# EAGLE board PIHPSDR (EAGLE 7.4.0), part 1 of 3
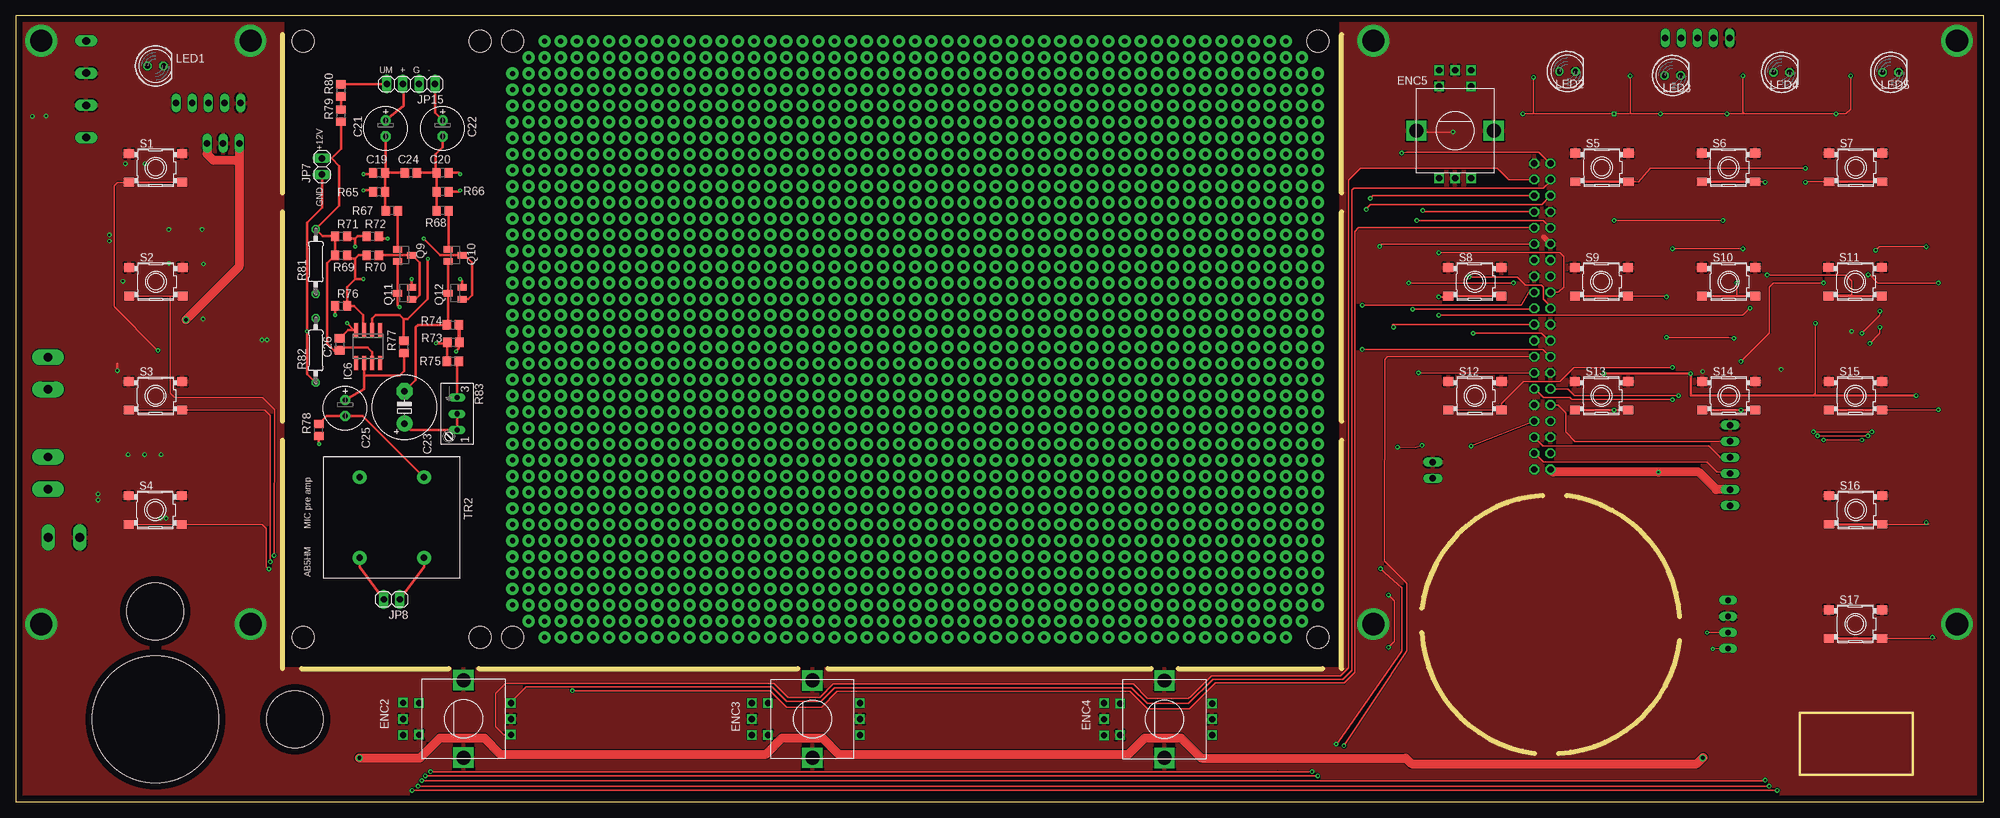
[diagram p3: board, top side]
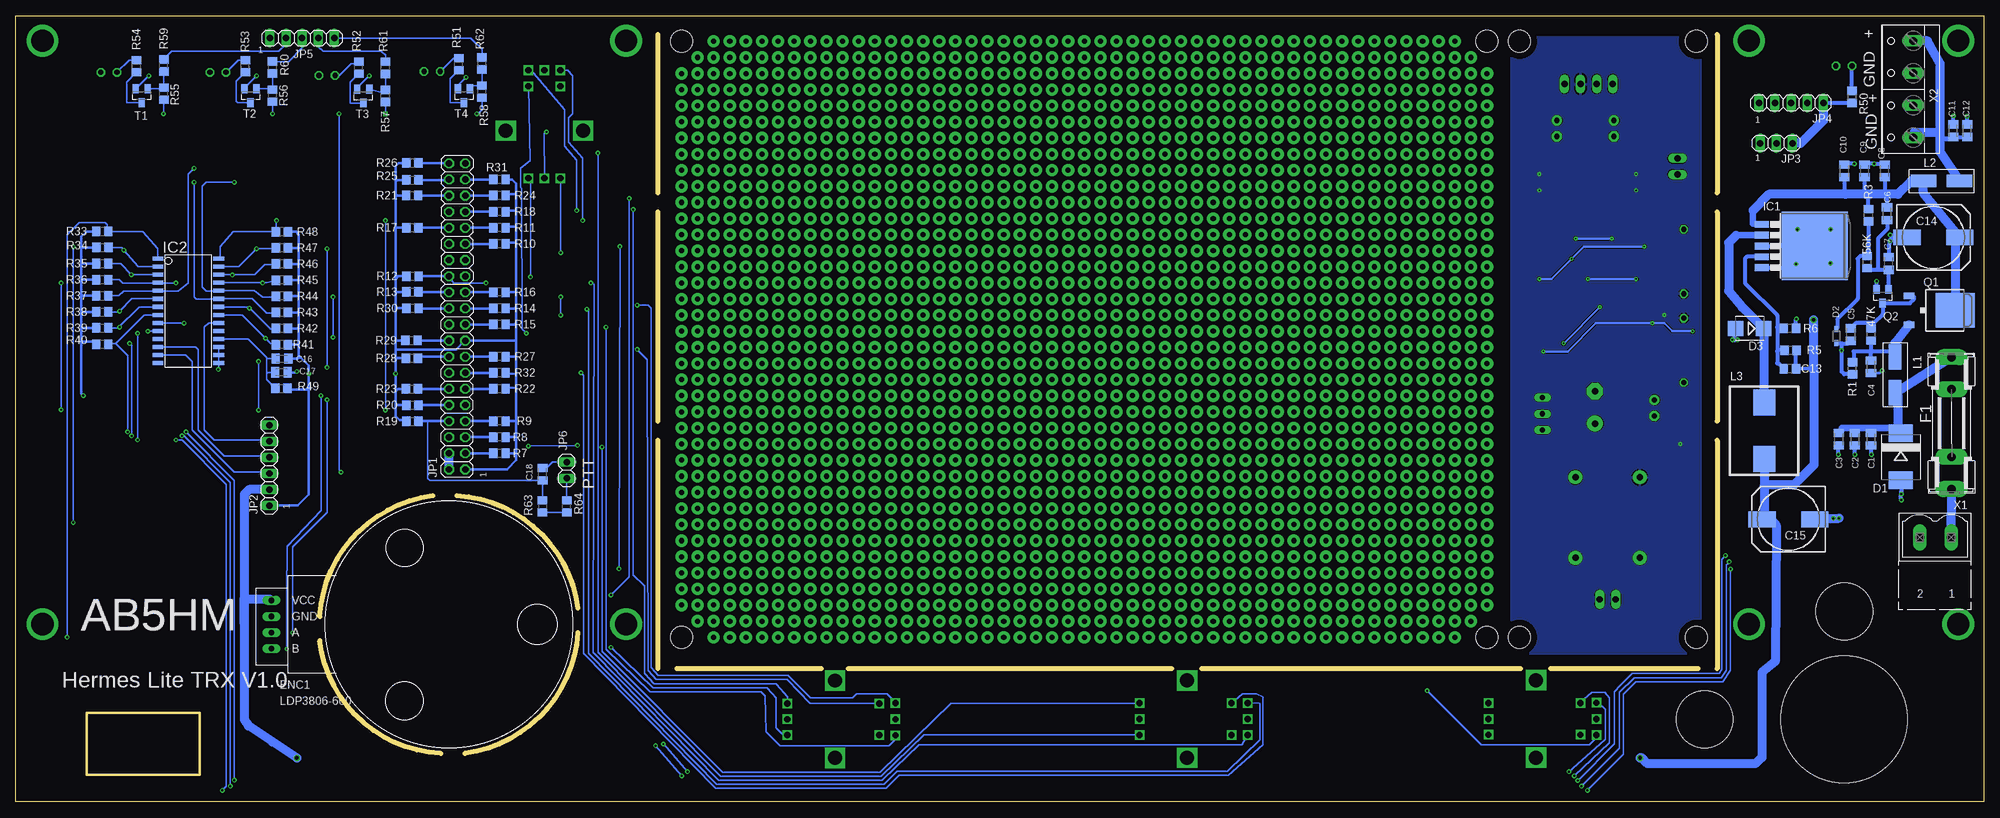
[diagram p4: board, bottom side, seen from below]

Size 310.21 x 123.94 mm. Coordinates in mm from the lower left corner, seen from the top.
Outline: 0,0 310.21,0 310.21,123.94 0,123.94 0,0
Copper layers (1*16): Top 0.035mm / dielectric 1.5mm / Bottom 0.035mm
Design rules "default *": minimum track width 10mil, minimum drill 0.19811875mm, track to track 4mil, track to pad 4mil, pad to pad 4mil, via to via 4mil, smd to smd 6mil, copper to edge 40mil, drill to drill 8mil, minimum pad ring 10mil, minimum via ring 8mil, stop-mask expansion 4mil, vias tented up to drill 0mil, thermal gap 10mil
Holes 9 mm at 22,30 44,13
Holes 20 mm at 22,13
Holes 3.5 mm at 45.26,119.92 73.2,119.92 78.28,119.92 205.28,119.92 205.28,25.94 78.28,25.94 73.2,25.94 45.26,25.94
Milling: 14 lines

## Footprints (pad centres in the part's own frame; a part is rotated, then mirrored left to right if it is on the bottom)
R0805 = smd 1.3 x 1.5: 1 -0.95,0; 2 0.95,0
C0805K = smd 1.3 x 1.6: 1 -1,0; 2 1,0
C0805 = smd 1.3 x 1.5: 1 -0.95,0; 2 0.95,0
140CLH-1010 = smd 4.3 x 2.5: + 4.15,0; - -4.15,0
E2,5-7 = drill 0.813 pad 1.6: + -1.27,0 | drill 0.813 pad 1.6 octagon: - 1.27,0
E5-10,5 = drill 1.016 pad 2.54: + -2.54,0 | drill 1.016 pad 2.54 octagon: - 2.54,0
SMC = smd 2.8 x 3.8: A 3.7,0; C -3.7,0
SOD323 = smd 1 x 0.6: 1 -1.1,0; 2 1.1,0
SMB = smd 2.4 x 2.4: A 2.2,0; C -2.2,0
LPD3806_ROTARY = drill 0.9 long: A -27.94,-1.27; B -27.94,-3.81; GND -27.94,1.27; VCC -27.94,3.81
ALPS_EC11E_SW = drill 1 square: A -2.5,-7.5; A' -2.54,9.525; B 2.5,-7.5; B' 2.54,9.525; C 0,-7.5; C' 0,9.525; D -2.5,7; E 2.5,7 | drill 2.2 square: GND1 -6.1,0; GND2 6.1,0
SHK20L = drill 1.321 pad 2.54 long: 1A -10.414,0; 1B -5.334,0; 2A 10.414,0; 2B 5.334,0
TO263-5 = smd 1.067 x 2.159: 1 -3.404,-5.791; 2 -1.702,-5.791; 3 0,-5.791; 4 1.702,-5.791; 5 3.404,-5.791 | smd 10.8 x 10.41: 6 0,2.54
SO28W = smd 0.65 x 1.7: 1 -7.62,-4.78; 2 -6.35,-4.78; 3 -5.08,-4.78; 4 -3.81,-4.78; 5 -2.54,-4.78; 6 -1.27,-4.78; 7 0,-4.78; 8 1.27,-4.78; 9 2.54,-4.78; 10 3.81,-4.78; 11 5.08,-4.78; 12 6.35,-4.78; 13 7.62,-4.78; 14 8.89,-4.78; 15 8.89,4.78; 16 7.62,4.78; 17 6.35,4.78; 18 5.08,4.78; 19 3.81,4.78; 20 2.54,4.78; 21 1.27,4.78; 22 0,4.78; 23 -1.27,4.78; 24 -2.54,4.78; 25 -3.81,4.78; 26 -5.08,4.78; 27 -6.35,4.78; 28 -7.62,4.78
SO8 = smd 0.6 x 2.2: 1 -1.905,-2.6; 2 -0.635,-2.6; 3 0.635,-2.6; 4 1.905,-2.6; 5 1.905,2.6; 6 0.635,2.6; 7 -0.635,2.6; 8 -1.905,2.6
2X20 = drill 1.016 octagon: 1 -24.13,-1.27; 2 -24.13,1.27; 3 -21.59,-1.27; 4 -21.59,1.27; 5 -19.05,-1.27; 6 -19.05,1.27; 7 -16.51,-1.27; 8 -16.51,1.27; 9 -13.97,-1.27; 10 -13.97,1.27; 11 -11.43,-1.27; 12 -11.43,1.27; 13 -8.89,-1.27; 14 -8.89,1.27; 15 -6.35,-1.27; 16 -6.35,1.27; 17 -3.81,-1.27; 18 -3.81,1.27; 19 -1.27,-1.27; 20 -1.27,1.27; 21 1.27,-1.27; 22 1.27,1.27; 23 3.81,-1.27; 24 3.81,1.27; 25 6.35,-1.27; 26 6.35,1.27; 27 8.89,-1.27; 28 8.89,1.27; 29 11.43,-1.27; 30 11.43,1.27; 31 13.97,-1.27; 32 13.97,1.27; 33 16.51,-1.27; 34 16.51,1.27; 35 19.05,-1.27; 36 19.05,1.27; 37 21.59,-1.27; 38 21.59,1.27; 39 24.13,-1.27; 40 24.13,1.27
1X06 = drill 1.016 long: 1 -6.35,0; 2 -3.81,0; 3 -1.27,0; 4 1.27,0; 5 3.81,0; 6 6.35,0
1X03 = drill 1.016 long: 1 -2.54,0; 2 0,0; 3 2.54,0
1X05 = drill 1.016 long: 1 -5.08,0; 2 -2.54,0; 3 0,0; 4 2.54,0; 5 5.08,0
1X02 = drill 1.016 long: 1 -1.27,0; 2 1.27,0
1X04 = drill 1.016 long: 1 -3.81,0; 2 -1.27,0; 3 1.27,0; 4 3.81,0
SM_BEAD = smd 4 x 2: P$1 -2.857,0; P$2 2.857,0
PULSE_PA4342 = smd 3.5 x 4.1: 1 0,4.445; 2 0,-4.445
LED5MM = drill 0.813 octagon: A -1.27,0; K 1.27,0
TO252 = smd 1 x 1.6: 1 -2.28,-4.8; 2 2.28,-4.8 | smd 5.4 x 6.2: 3 0,2.5
SOT23 = smd 1 x 1.4: 1 -0.95,-1.1; 2 0.95,-1.1; 3 0,1.1
SOT23-BEC = smd 1 x 1.4: B -0.95,-1.1; C 0,1.1; E 0.95,-1.1
0207/10 = drill 0.813 octagon: 1 -5.08,0; 2 5.08,0
S64W = drill 0.813 long: A 2.54,1.27; E -2.54,1.27; S 0,1.27
TL3301-SMD = smd 1.6 x 1.4: 1 -4.2,2.25; 2 4.2,2.25; 3 -4.2,-2.25; 4 4.2,-2.25
SV1-500 = drill 1 pad 2.184: 1 -5.08,-6.35; 3 5.08,-6.35; 4 5.08,6.35; 6 -5.08,6.35
MSTBV2 = drill 1.397 long: 1 -2.5,0; 2 2.5,0
W237-4P = drill 1.194 long: 1 -7.62,-0.635; 2 -2.54,-0.635; 3 2.54,-0.635; 4 7.62,-0.635

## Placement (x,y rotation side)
47K  100k  [R0805]  17.76,73.68 270 bottom
56K  180k  [R0805]  18.39,85.11 270 bottom
C1  10u  [C0805K]  17.76,57.17 270 bottom
C2  10u  [C0805K]  20.3,57.17 270 bottom
C3  0.1u  [C0805K]  22.84,57.17 270 bottom
C4  10u  [C0805K]  17.76,68.6 270 bottom
C5  0.1u  [C0805K]  20.93,73.68 270 bottom
C6  10u  [C0805K]  15.22,92.73 270 bottom
C7  0.1u  [C0805K]  14.98,84.88 90 bottom
C8  10u  [C0805K]  15.61,99.48 90 bottom
C9  0.1u  [C0805K]  18.79,99.48 90 bottom
C10  0.1u  [C0805K]  21.96,99.48 90 bottom
C11  0.1u  [C0805K]  4.82,105.83 90 bottom
C12  0.1u  [C0805K]  2.59,105.83 90 bottom
C13  np  [C0805]  30.54,68.29 180 bottom
C14  220u  [140CLH-1010]  7.91,89 0 bottom
C15  220u  [140CLH-1010]  30.77,44.55 180 bottom
C16  10u  [C0805K]  268.26,69.88 180 bottom
C17  1n  [C0805K]  268.35,67.73 0 bottom
C18  100n  [C0805K]  227.19,51.66 90 bottom
C19  680p  [C0805]  57.27,99.19 180 top
C20  680p  [C0805]  67.27,99.19 180 top
C21  47/63  [E2,5-7]  58.27,106.19 270 top
C22  47/63  [E2,5-7]  67.27,106.19 270 top
C23  1000/6  [E5-10,5]  61.27,62.19 90 top
C24  330p  [C0805]  62.27,99.19 180 top
C25  47/63  [E2,5-7]  51.91,62.09 270 top
C26  0.1u  [C0805]  51.05,72.13 270 top
D1  [SMC]  13.07,54.4 270 bottom
D2  BAS16J  [SOD323]  23.23,73.45 90 bottom
D3  SS54B-HF  [SMB]  36.89,74.64 180 bottom
ENC1  LDP3806-600  [LPD3806_ROTARY]  241.96,27.96 0 bottom
ENC2  EC11E_SW  [ALPS_EC11E_SW]  70.57,13.07 90 top
ENC3  EC11E_SW  [ALPS_EC11E_SW]  125.57,13.04 90 top
ENC4  EC11E_SW  [ALPS_EC11E_SW]  181.07,13.01 90 top
ENC5  EC11E_SW  [ALPS_EC11E_SW]  226.89,105.84 0 top
F1  5A  [SHK20L]  5.06,59.71 90 bottom
IC1  LM2596S  [TO263-5]  29.19,87.65 270 bottom
IC2  MCP23017SO  [SO28W]  283.03,78.05 270 bottom
IC6  TL071  [SO8]  55.54,71.83 180 top
JP1  [2X20]  240.65,76.54 90 bottom
JP2  [1X06]  270.25,53.04 90 bottom
JP3  [1X03]  32.67,103.85 180 bottom
JP4  [1X05]  30.34,110.2 180 bottom
JP5  [1X05]  265.08,120.43 0 bottom
JP6  PTT  [1X02]  223.38,52.29 90 bottom
JP7  [1X02]  48.27,100.19 90 top
JP8  [1X02]  59.27,31.92 180 top
JP15  [1X04]  62.27,113.19 180 top
L1  2743021447  [SM_BEAD]  13.95,67.33 90 bottom
L2  2743021447  [SM_BEAD]  6.64,97.89 0 bottom
L3  47uH  [PULSE_PA4342]  34.58,58.52 0 bottom
LED1  [LED5MM]  22.02,116.04 0 top
LED2  [LED5MM]  244.59,115.17 0 top
LED3  [LED5MM]  261.16,114.53 0 top
LED4  [LED5MM]  278.36,115.03 0 top
LED5  [LED5MM]  295.55,115.03 0 top
Q1  FDD6685  [TO252]  6.96,77.49 270 bottom
Q2  IRLM6244  [SOT23]  15.93,79.72 180 bottom
Q9  BC847A  [SOT23]  61.27,86.19 270 top
Q10  BC847A  [SOT23]  69.27,86.19 270 top
Q11  BC858A  [SOT23-BEC]  61.27,80.19 90 top
Q12  BC858A  [SOT23-BEC]  69.27,80.19 90 top
R1  10k  [R0805]  20.69,68.37 90 bottom
R3  100k  [R0805]  18.15,92.5 90 bottom
R5  3K05  [R0805]  30.45,71.22 0 bottom
R6  1k  [R0805]  30.54,74.64 180 bottom
R7  10k  [R0805]  233.97,54.95 180 bottom
R8  10k  [R0805]  233.97,57.49 180 bottom
R9  10k  [R0805]  233.97,60.03 180 bottom
R10  10k  [R0805]  233.97,87.97 180 bottom
R11  10  [R0805]  233.97,90.52 180 bottom
R12  10k  [R0805]  247.68,82.89 0 bottom
R13  10k  [R0805]  247.69,80.4 0 bottom
R14  10k  [R0805]  233.97,77.81 180 bottom
R15  10k  [R0805]  233.97,75.28 180 bottom
R16  10k  [R0805]  233.97,80.36 180 bottom
R17  10k  [R0805]  247.71,90.54 0 bottom
R18  10k  [R0805]  233.97,93.06 180 bottom
R19  10k  [R0805]  247.71,60 0 bottom
R20  10k  [R0805]  247.71,62.57 0 bottom
R21  10k  [R0805]  247.73,95.62 0 bottom
R22  10k  [R0805]  233.97,65.11 180 bottom
R23  10k  [R0805]  247.77,65.11 0 bottom
R24  10k  [R0805]  233.97,95.59 180 bottom
R25  10k  [R0805]  247.71,98.05 0 bottom
R26  10k  [R0805]  247.71,100.75 0 bottom
R27  10k  [R0805]  233.97,70.19 180 bottom
R28  10k  [R0805]  247.79,69.95 0 bottom
R29  10k  [R0805]  247.84,72.74 0 bottom
R30  10k  [R0805]  247.68,77.82 0 bottom
R31  10k  [R0805]  233.97,98.14 180 bottom
R32  10k  [R0805]  233.97,67.66 180 bottom
R33  10k  [R0805]  296.61,89.95 0 bottom
R34  10k  [R0805]  296.56,87.41 0 bottom
R35  10k  [R0805]  296.61,84.87 0 bottom
R36  10k  [R0805]  296.61,82.33 0 bottom
R37  10k  [R0805]  296.61,79.79 0 bottom
R38  10k  [R0805]  296.61,77.25 0 bottom
R39  10k  [R0805]  296.61,74.71 0 bottom
R40  10k  [R0805]  296.61,72.17 0 bottom
R41  10k  [R0805]  268.26,72.1 180 bottom
R42  10k  [R0805]  268.26,74.64 180 bottom
R43  10k  [R0805]  268.26,77.18 180 bottom
R44  10k  [R0805]  268.26,79.72 180 bottom
R45  10k  [R0805]  268.26,82.26 180 bottom
R46  10k  [R0805]  268.26,84.8 180 bottom
R47  10k  [R0805]  268.26,87.34 180 bottom
R48  10k  [R0805]  268.26,89.88 180 bottom
R49  [R0805]  268.35,65.19 0 bottom
R50  1k5  [R0805]  20.77,111.14 270 bottom
R51  470R  [R0805]  240.4,116.31 90 bottom
R52  470R  [R0805]  256.16,115.78 90 bottom
R53  470R  [R0805]  274.06,116 90 bottom
R54  470R  [R0805]  291.2,116 90 bottom
R55  10k  [R0805]  286.88,111.67 90 bottom
R56  [R0805]  269.73,111.35 90 bottom
R57  [R0805]  251.95,111.3 90 bottom
R58  [R0805]  236.71,111.98 90 bottom
R59  39k  [R0805]  286.88,116.11 90 bottom
R60  39k  [R0805]  269.73,115.79 90 bottom
R61  39k  [R0805]  251.95,115.75 90 bottom
R62  39k  [R0805]  236.71,116.43 90 bottom
R63  1k  [R0805]  227.19,46.58 270 bottom
R64  1k Ferrite  [R0805]  223.38,46.58 90 bottom
R65  1k2  [R0805]  57.27,96.19 0 top
R66  1k2  [R0805]  67.27,96.19 180 top
R67  10  [R0805]  59.27,93.19 180 top
R68  10  [R0805]  67.27,93.19 180 top
R69  680  [R0805]  51.27,86.19 0 top
R70  680  [R0805]  56.27,86.19 0 top
R71  680  [R0805]  51.27,89.17 0 top
R72  680  [R0805]  56.27,89.19 0 top
R73  2k2  [R0805]  68.97,72.47 0 top
R74  2k2  [R0805]  68.89,75.19 0 top
R75  150  [R0805]  68.91,69.46 180 top
R76  150k  [R0805]  51.27,78.19 0 top
R77  150k  [R0805]  61.17,71.73 90 top
R78  10k  [R0805]  47.76,58.63 90 top
R79  10k  [R0805]  51.27,108.19 90 top
R80  1k Ferr.  [R0805]  51.27,112.19 90 top
R81  [0207/10]  47.27,85.19 90 top
R82  [0207/10]  47.27,71.19 90 top
R83  100k  [S64W]  68.27,61.19 270 top
S1  TL3301  [TL3301-SMD]  22.04,99.97 0 top
S2  [TL3301-SMD]  22.07,82.01 0 top
S3  [TL3301-SMD]  22.02,64.01 0 top
S4  [TL3301-SMD]  21.96,46.01 0 top
S5  [TL3301-SMD]  250.03,100.01 0 top
S6  [TL3301-SMD]  269.98,100.01 0 top
S7  [TL3301-SMD]  290.05,100.01 0 top
S8  [TL3301-SMD]  230,82.01 0 top
S9  [TL3301-SMD]  249.94,82.01 0 top
S10  [TL3301-SMD]  270.01,82.01 0 top
S11  [TL3301-SMD]  289.95,82.03 0 top
S12  [TL3301-SMD]  230.02,64.03 0 top
S13  [TL3301-SMD]  249.97,64.03 0 top
S14  [TL3301-SMD]  270.04,64.03 0 top
S15  [TL3301-SMD]  289.98,64.03 0 top
S16  [TL3301-SMD]  290.05,46.02 0 top
S17  [TL3301-SMD]  290,28.02 0 top
T1  [SOT23]  290.37,111.35 180 bottom
T2  [SOT23]  273.23,111.35 180 bottom
T3  [SOT23]  255.44,111.3 180 bottom
T4  [SOT23]  239.57,111.35 180 bottom
TR2  SV1-500  [SV1-500]  59.27,44.83 180 top
X1  [MSTBV2]  7.59,41.69 180 bottom
X2  [W237-4P]  11.73,112.37 90 bottom

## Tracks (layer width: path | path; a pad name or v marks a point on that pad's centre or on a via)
+3V3  (via drill 0.3)
  Top 0.254: v283.7,75.47 283.7,64.36 283.38,64.04
  Top 0.406: v250.37,67.53 v264.02,67.53 264.02,64.04 283.38,64.04 v299.58,64.04
  Bottom 0.254: IC2.9 283.75,75.51 v283.7,75.47
  Bottom 0.305: R22.1 232.82,65.31 231.31,65.31 | R32.1 232.9,67.53 231.31,67.53
  Bottom 0.406: R31.1 231.95,98.14 231.31,97.5 231.31,95.79 | 231.31,95.79 231.31,93.25 | 231.31,93.25 231.31,90.71 | 231.31,90.71 231.31,88.17 | 231.31,88.17 231.31,80.55 | 231.31,80.55 231.31,78.01 | 231.31,78.01 231.31,75.47 | 231.31,75.47 231.31,72.93 | 231.31,72.93 231.31,70.39 | 231.31,70.39 231.31,67.53 231.31,65.31 231.31,60.23 | 231.31,60.23 231.31,57.69 | 231.31,57.69 231.31,55.15 | 231.31,55.15 231.31,53.88 232.79,52.41 JP1.1 | R24.1 232.82,95.79 231.31,95.79 | R18.1 232.82,93.25 231.31,93.25 | R11.1 232.82,90.71 231.31,90.71 | R10.1 232.82,88.17 231.31,88.17 | R16.1 231.51,80.36 231.31,80.55 | R14.1 231.51,77.81 231.31,78.01 | R15.1 231.51,75.28 231.31,75.47 | R27.1 231.51,70.19 231.31,70.39 | 231.31,72.93 231.52,72.73 JP1.17 239.46,72.73 240.84,71.34 250.37,71.34 | R9.1 231.51,60.03 231.31,60.23 | R8.1 231.51,57.49 231.31,57.69 | R7.1 231.51,54.95 231.31,55.15 | R26.1 249.85,100.75 250.37,100.23 250.37,97.69 | 250.37,97.69 250.37,95.79 | 250.37,95.79 250.37,90.71 | 250.37,90.71 250.37,82.45 | 250.37,82.45 250.37,80.55 | 250.37,80.55 250.37,78.01 | 250.37,78.01 250.37,72.93 | 250.37,72.93 250.37,71.34 | 250.37,71.34 250.37,69.75 | 250.37,69.75 v250.37,67.53 250.37,64.67 | 250.37,64.67 250.37,62.77 | 250.37,62.77 250.37,60.87 249.73,60.23 248.89,60.23 R19.1 | R25.1 250.01,98.05 250.37,97.69 | R21.1 250.19,95.62 250.37,95.79 | R17.1 250.19,90.54 250.37,90.71 | R12.1 249.93,82.89 250.37,82.45 | R13.1 250.21,80.4 250.37,80.55 | R30.1 250.18,77.82 250.37,78.01 | R29.1 250.18,72.74 250.37,72.93 | R23.1 249.93,65.11 250.37,64.67 | R20.1 250.16,62.57 250.37,62.77 | R28.1 250.17,69.95 250.37,69.75 | R48.1 266.05,89.88 265.61,89.44 265.61,87.53
  Bottom 0.406: 265.61,87.53 265.61,84.68 | 265.61,84.68 265.61,82.45 | 265.61,82.45 265.61,79.6 | 265.61,79.6 265.61,77.38 | 265.61,77.38 265.61,74.83 | 265.61,74.83 265.61,71.98 | 265.61,71.98 265.61,70.07 | 265.61,70.07 265.29,70.07 264.02,68.8 v264.02,67.53 264.02,65.31 | 264.02,65.31 264.33,64.99 267.2,64.99 R49.2 | R47.1 265.8,87.34 265.61,87.53 | R46.1 265.73,84.8 265.61,84.68 | R45.1 265.8,82.26 265.61,82.45 | R44.1 265.73,79.72 265.61,79.6 | R43.1 265.8,77.18 265.61,77.38 | R42.1 265.8,74.64 265.61,74.83 | R41.1 265.73,72.1 265.61,71.98 | C16.1 265.8,69.88 265.61,70.07 | R33.1 299.06,89.95 299.89,89.12 299.89,87.22 | 299.89,87.22 299.89,85 | 299.89,85 299.89,82.45 | 299.89,82.45 299.89,79.6 | 299.89,79.6 299.89,77.06 | 299.89,77.06 299.89,74.83 | 299.89,74.83 299.89,72.3 | 299.89,72.3 299.89,64.36 v299.58,64.04 | R34.1 299.7,87.41 299.89,87.22 | R35.1 299.77,84.87 299.89,85 | R36.1 299.77,82.33 299.89,82.45 | R37.1 299.7,79.79 299.89,79.6 | R38.1 299.7,77.25 299.89,77.06 | R39.1 299.77,74.71 299.89,74.83 | R40.1 297.56,72.5 297.67,72.61 299.58,72.61 299.89,72.3 | JP2.1 265.81,46.69 264.02,48.48 264.02,65.31
+5V  (via drill 0.3, 0.6)
  Top 0.254: 272.5,108.49 v286.94,108.49 288.5,108.49 289.25,109.24 v289.25,114.5 | 272.5,108.49 v269.73,108.49 v259.25,108.49 254.5,108.49 | 254.5,108.49 v251.95,108.49 239.25,108.49 | 239.25,108.49 v237.57,108.49 | v239.25,114.25 239.25,108.49 | v254.5,114.5 254.5,108.49 | v272.25,114.5 272.25,108.74 272.5,108.49
  Top 0.61: 35.13,101.17 35.2,101.1
  Top 1.422: v54.15,6.92 63.7,6.92 66.85,10.06 73.83,10.06 76.38,7.53 118.28,7.53 120.83,10.06 127.18,10.06 129.72,7.53 175.44,7.53 177.97,10.06 183.69,10.06 186.87,6.89 219.11,6.89 220,6 265,6 266,7 v265.92,6.92 | JP3.1 30.13,102.15 31.12,101.17 35.13,101.17 | 35.2,101.1 35.2,100.67 | 35.2,100.67 35.2,84.39 v26.82,76.01 | JP3.3 35.22,100.69 35.2,100.67 | JP2.2 268.03,49.23 265.29,51.98 v258.94,51.98 242.35,51.98 JP1.2
  Bottom 0.254: v237.57,108.49 237.35,108.49 236.71,109.12 R58.1 | R55.1 286.88,108.81 v286.94,108.49 | R56.1 v269.73,108.49 | R57.1 v251.95,108.49 | v259.25,108.49 259.25,52.29 v258.94,51.98 | T4.2 240.52,112.98 v239.25,114.25 | T3.2 256.39,112.61 v254.5,114.5 | T2.2 274.18,112.58 v272.25,114.5 | T1.2 291.3,112.45 v289.25,114.5
  Bottom 0.406: ENC1.VCC 270.07,31.77 270.25,31.95
  Bottom 0.61: 26.7,67.92 26.7,68.24 C13.1 29.59,71.13 R5.2 | R50.2 JP4.1
  Bottom 1.422: L3.2 34.58,49.77 | 34.58,49.77 34.58,44.89 C15.+ arc90 32.67,43.38 32.88,22.13 34.95,20.37 34.95,7 35,7 36,6 53,6 54,7 v54.15,6.92 | 34.58,49.77 34.41,49.94 29.94,49.94 26.7,53.18 26.7,67.92 26.82,68.03 v26.82,76.01 | JP4.1 25.26,107.42 28.86,103.83 30.11,103.83 JP3.1 | JP1.2 JP1.4 | JP2.2 273.43,49.23 274.18,48.48 274.18,24.04 | 274.18,24.04 274.18,12.97 273.54,11.97 269.76,9.43 v265.92,6.92 | 270.25,31.95 274.26,31.95 274.18,24.04
+12V
  Top 0.406: JP7.2 49.75,101.46 | 49.75,101.46 50.98,100.23 50.98,93.97 R81.2 48.37,89.17 R71.1 R69.1 49.07,84.94 49.07,72.3 50.19,71.18 C26.2 51.52,71.66 55.42,71.66 56.17,70.91 IC6.7 | R79.1 51.27,102.98 49.75,101.46
-12V  (via drill 0.2)
  Top 0.406: JP7.1 48.27,93.72 45.9,91.34 v45.9,74.2 45.9,67.48 R82.1 | R73.2 69.92,75.11 R74.2 69.84,71.47 v69.39,71.03 | C26.1 52.39,74.42 IC6.4 53.29,74.42 v52.24,75.47
  Bottom 0.406: v45.9,74.2 49.07,74.2 50.34,75.47 v52.24,75.47 61.14,75.47 65.58,71.03 v69.39,71.03
GND  (via drill 0.3, 3.5 pad 5)
  Top 0.254: v226.55,105.63 220.75,105.63 ENC5.GND1 | JP1.30 241.91,88.05 | v289.42,74.2 289.74,74.2
  Top 0.406: v16,68 16,69
  Top 0.813: 241.91,88.05 240.84,89.12
  Bottom 0.254: IC2.17 IC2.16 IC2.15 278.25,68.22 v278.31,68.17 | ENC5.C 226.96,105.39 v226.55,105.63 | IC2.10 289.69,74.24 v289.42,74.2 | C18.2 226.5,52.66 225.6,53.56 JP6.2
  Bottom 0.406: C17.2 266.05,67.73 v265.92,67.85 | C4.2 16.4,67.6 v16,68
  Bottom 0.61: Q2.2 16.89,82.06 v16.86,82.09 | v38.8,72.83 39.58,72.83 39.61,72.8 39.26,72.8 39.19,72.87 39.19,74.54 D3.A | C14.- 13.08,89 v14.72,89.37 | v14.72,88.42 13.45,89.19 13.35,89.29 14.73,88.65 14.99,87.75 14.99,85.9 C7.2 | C11.2 4.82,108.11 v4.78,108.15 | C12.2 v2.6,108.1 | C8.2 15.73,100.61 v17.24,100.61 18.66,100.61 C9.2 | v20.39,100.61 21.84,100.61 C10.2 | IC1.6 26.65,87.71 v24.11,90.25 | IC1.3 31.96,87.65 v29.36,90.25 | IC1.5 30.12,84.25 v29.58,84.79 | R6.1 29.59,76.08 v29.52,76.14 | v12.97,47.57 13.05,47.88 13,48.89 12.91,48.89 12.94,48.86 12.94,50.57 D1.A | v17.69,54.74 17.69,56.1 C1.2 | v20.29,54.74 C2.2 | v22.89,54.75 22.89,56.12 C3.2
  Bottom 1.422: C15.- 25.98,44.71 v22.82,44.7
  other vias: 39.61,72.85 23.69,44.7 12.97,48.52 24.17,84.94 4,120 37,120 4,28 37,28 214,120 306,120 214,28 306,28
  pour Top: -1.73,126.27 42,126.27 42,21 209,21 209,126 311.96,126.27 311.96,-0.73 -1.73,-0.73
GND1  (via drill 0.2)
  Top 0.406: v54.78,98.97 56.09,98.97 C19.2 | v54.78,96.42 56.09,96.42 R65.1 | C20.1 69.8,99.19 v70.03,98.97 | R66.1 69.79,96.19 v70.03,96.42 | v50.34,76.74 50.34,78.17 R76.1 | R78.1 47.76,56.46 v47.8,56.42
  pour Bottom: 44.62,120.56 74.47,120.56 74.47,23.4 44.62,23.4
GPA0  (via drill 0.3)
  Top 0.254: S9.4 260.05,79.76 v260.21,79.6 | v260.21,73.25 270.05,73.25 v270.84,73.09
  Top 0.406: S9.3 S9.4
  Bottom 0.254: IC2.21 274.54,76.78 v270.84,73.09 270.05,72.3 269.4,72.3 R41.2 | v260.21,79.6 v260.21,73.25
GPA1  (via drill 0.3)
  Top 0.254: S8.4 225.76,79.76 225.6,79.6 v224.33,79.6 | v224.33,76.74 272.27,76.74 v273.38,77.85
  Top 0.406: S8.3 S8.4
  Bottom 0.254: IC2.22 274.22,78.05 274.18,78.01 273.86,78.01 | 273.86,78.01 273.54,78.01 v273.38,77.85 | v273.38,77.85 270.05,74.52 269.33,74.52 R42.2 | v224.33,79.6 v224.33,76.74 | v273.38,77.85 273.7,77.85 273.86,78.01
GPA2  (via drill 0.3)
  Top 0.254: S7.3 282.18,97.76 v282.12,97.69
  Top 0.406: S7.3 S7.4
  Bottom 0.254: R43.2 269.33,77.06 270.69,77.06 272.95,79.32 IC2.23 278.3,79.28 281.8,79.28 282.12,79.6 v282.12,97.69
GPA3  (via drill 0.3)
  Top 0.254: S6.4 275.7,97.76 v275.76,97.69
  Top 0.406: S6.3 S6.4
  Bottom 0.254: R44.2 269.33,79.6 271.32,79.6 272.63,80.59 IC2.24 278.3,80.55 280.21,80.55 280.85,81.19 280.85,97.06 280.21,97.69 v275.76,97.69
GPA4  (via drill 0.3)
  Top 0.254: v271.32,81.82 271.32,79.76
  Top 0.406: S10.4 271.32,79.76 S10.3
  Bottom 0.254: IC2.25 271.28,81.86 | R45.2 270.56,81.86 271.28,81.86 | 271.28,81.86 v271.32,81.82
GPA5  (via drill 0.3)
  Top 0.254: v276.08,83.09 288.46,83.09 289.42,82.14 289.42,79.92 285.61,79.92 S11.3
  Top 0.406: S11.4 S11.3
  Bottom 0.254: R46.2 269.33,84.68 271,84.68 272.55,83.13 IC2.26 276.13,83.13 v276.08,83.09
GPA6  (via drill 0.3)
  Top 0.254: S12.3 S12.4 234.22,62.82 237.66,66.26 243.38,66.26 245.6,68.48 v261.16,68.48 | v261.16,87.22 v272.27,87.22
  Bottom 0.254: IC2.27 275.09,84.4 v272.27,87.22 269.33,87.22 R47.2 | v261.16,68.48 v261.16,87.22
GPA7  (via drill 0.3)
  Top 0.254: v269.1,91.66 v251.95,91.66
  Top 0.406: S13.4 v251.95,61.77 S13.3
  Bottom 0.254: IC2.28 277.99,85.94 277.99,87.53 275.96,89.88 R48.2 269.21,91.55 v269.1,91.66 | v251.95,91.66 v251.95,61.77
GPB0  (via drill 0.3)
  Top 0.254: S17.3 302.59,25.77 v302.12,25.94
  Top 0.406: S17.4 S17.3
  Bottom 0.254: IC2.1 287.83,85.69 287.83,87.22 290.25,89.95 R33.2 295.77,90.06 295.77,91.03 296.08,91.34 300.21,91.34 302.12,89.44 v302.12,25.94
GPB1  (via drill 0.3)
  Top 0.254: S16.3 301.54,43.77 v301.17,44.04 | v301.17,87.53 293.75,87.53 v293.18,86.97
  Top 0.406: S16.4 S16.3
  Bottom 0.254: IC2.2 290.89,84.4 v293.18,86.97 | v293.18,86.97 293.47,87.29 | 293.47,87.29 293.55,87.38 295.57,87.38 R34.2 | v301.17,44.04 v301.17,87.53 | v293.18,86.97 293.18,87.01 293.47,87.29
GPB2  (via drill 0.3)
  Top 0.254: v292,83.13 292.23,83.13 293.55,81.82 v303.07,81.82 | v303.07,61.82 294.22,61.82 S15.4
  Top 0.406: S15.4 S15.3
  Bottom 0.254: IC2.3 v292,83.13 293.7,84.84 295.62,84.84 R35.2 | v303.07,81.82 v303.07,61.82
GPB3  (via drill 0.3)
  Top 0.254: v284.97,81.82 277.04,81.82 276.4,81.19 276.4,73.88 v271.95,69.44
  Top 0.406: S14.4 v271.95,61.77 S14.3
  Bottom 0.254: R36.2 293.9,82.33 293.39,81.82 287.86,81.82 | 287.86,81.82 IC2.4 | 287.86,81.82 v284.97,81.82 | v271.95,69.44 v271.95,61.77
GPB4  (via drill 0.3)
  Top 0.254: S5.4 255.38,97.76 255.76,97.69 257.67,99.92 v282.12,99.92
  Top 0.406: S5.3 S5.4
  Bottom 0.254: R37.2 293.99,79.79 293.23,80.55 287.86,80.55 IC2.5 287.77,80.55 284.65,80.55 283.07,81.82 283.07,98.97 v282.12,99.92
GPB5  (via drill 0.3)
  Top 0.254: S4.3 S4.4 38.8,43.76 39.47,43.09 39.47,37.05 v39.9,36.72 | v62.46,1.8 v277.67,1.8 | v293.86,77.38 293.86,76.74 v291,73.88 | v291,57.05 v284.97,57.05
  Bottom 0.254: IC2.6 291.91,79.32 v293.86,77.38 294.02,77.22 295.62,77.22 R38.2 | v39.9,36.72 39.9,20.76 41.08,18.95 54.81,18.95 56.79,16.97 56.79,7.47 v62.46,1.8 | v291,73.88 v291,57.05 | v284.97,57.05 284.02,57.05 277.04,50.07 277.04,2.43 v277.67,1.8
GPB6  (via drill 0.3)
  Top 0.254: S3.3 S3.4 39.24,61.76 40.09,60.91 40.09,37.86 | 40.09,37.86 40.09,37.84 | 40.09,37.86 v40.11,37.84 | v63.39,2.46 v276.4,2.46 | v293.86,74.83 293.86,73.88 v292.27,72.3 | v291.96,57.69 v284.02,57.69
  Bottom 0.254: IC2.7 290.8,78.05 294.18,74.68 | 294.18,74.68 295.62,74.68 R39.2 | v40.11,37.84 40.11,37.71 40.57,37.37 40.57,20.71 41.33,19.58 55.09,19.58 57.44,17.23 57.44,8.41 v63.39,2.46 | 294.18,74.68 294.02,74.68 v293.86,74.83 | v292.27,72.3 291.96,71.98 v291.96,57.69 | v284.02,57.69 283.7,57.69 276.4,50.39 v276.4,2.46
GPB7  (via drill 0.3)
  Top 0.254: S2.3 24.34,79.76 | 24.34,79.76 S2.4 | v40.71,38.84 40.79,61.86 38.91,63.74 25.07,63.74 24.34,64.47 24.34,79.76 | v63.98,3.34 275.71,3.34 v275.76,3.4 | v283.38,58.33 v292.59,58.33
  Bottom 0.254: IC2.8 290.01,76.78 294.5,72.3 | 294.5,72.3 295.53,72.3 R40.2 | v40.71,38.84 41.28,38.2 41.28,20.89 41.67,20.25 51.21,20.25 51.24,20.27 55.36,20.27 57.45,18.19 58.09,17.48 58.19,17.38 58.19,9.13 v63.98,3.34 | v275.76,3.4 275.76,50.7 v283.38,58.33 | v292.59,58.33 292.59,70.39 294.5,72.3
GPIO2
  Top 0.254: JP1.3 239.46,54.95 240.84,53.56 266.56,53.56 268.14,51.98 270.04,51.98 JP2.3
  Bottom 0.254: IC2.13 283.43,70.43 282.43,69.44 282.43,58.64 275.76,51.98 270.45,51.98 JP2.3
  Bottom 0.406: JP1.3 R7.2
GPIO3
  Top 0.254: JP2.4 268.67,54.31 266.88,56.1 240.76,56.1 JP1.5
  Bottom 0.254: IC2.12 281.84,71.7 281.48,71.34 281.48,58.64 277.35,54.52 270.45,54.52 JP2.4
  Bottom 0.406: R8.2 239.37,57.49 JP1.5
GPIO4  (via drill 0.3)
  Top 0.254: v217.82,55.94 220.63,55.9 v221.68,56.22 | v229.41,56.1 JP1.7
  Bottom 0.254: ENC3.B 162.82,15.54 174.01,4.67 198.77,4.67 217.82,23.72 v217.82,55.94 | v221.68,56.22 v229.41,56.1
  Bottom 0.406: R9.2 239.37,60.03 JP1.7
GPIO5  (via drill 0.3)
  Top 0.254: v65.37,4.75 198.92,4.75 v204.32,4.74 | v208.13,9.11 208.46,9.43 218.49,23.81 218.49,33.69 v215.12,36.73 | v214.99,87.58 215.38,87.97 JP1.29
  Bottom 0.254: ENC2.B' 60.71,15.61 59.67,14.57 59.67,9.85 60.47,9.05 v65.37,4.75 | v204.32,4.74 v208.13,9.11 | v215.12,36.73 v214.99,87.58
  Bottom 0.406: JP1.29 R10.2
GPIO6  (via drill 0.3)
  Top 0.254: v87.72,17.52 118.89,17.52 121.48,14.93 127.04,14.93 129.49,17.38 175.67,17.38 178.36,14.69 185.03,14.69 189.08,18.75 209.44,18.73 211.09,20.41 211.09,89.94 211.66,90.51 JP1.31
  Bottom 0.254: ENC2.A' 61.05,10.12 62.15,9.01 79.21,9.01 v87.72,17.52
  Bottom 0.406: JP1.31 234.92,90.51 R11.2
GPIO7  (via drill 0.3)
  Top 0.254: v219.57,81.82 v236.08,81.82
  Bottom 0.254: ENC3.A' 116.9,8.95 167.81,8.95 173.53,3.56 173.69,3.4 199.41,3.4 219.25,23.56 219.09,81.66 v219.57,81.82 | v236.08,81.82 241.16,81.82 JP1.26
  Bottom 0.406: R12.2 JP1.26
GPIO8  (via drill 0.3)
  Top 0.254: JP1.24 243.18,80.35 244.01,81.19 244.01,85.95 243.38,86.58 v224.33,86.58
  Bottom 0.254: v224.33,86.58 224.33,98.15 ENC5.A
  Bottom 0.406: R13.2 241.96,80.4 JP1.24
GPIO9  (via drill 0.3)
  Top 0.254: v220.2,77.69 239.26,77.69 JP1.21
  Bottom 0.254: ENC3.B' 114.11,15.49 114.11,9.77 119.24,4.83 171.31,4.83 173.37,2.76 199.72,2.76 219.88,23.4 219.88,77.38 v220.2,77.69
  Bottom 0.305: JP1.21 239.37,77.81
  Bottom 0.406: 239.37,77.81 R14.2
GPIO10  (via drill 0.3)
  Top 0.254: v217.19,74.83 216.98,75.27 JP1.19
  Bottom 0.254: ENC4.A' 171.54,9.83 172.58,8.79 189.72,8.79 191.94,11.02 192.1,16.73 192.74,17.37 210.2,17.37 217.19,24.04 v217.19,74.83
  Bottom 0.305: JP1.19 239.37,75.28
  Bottom 0.406: 239.37,75.28 R15.2
GPIO11  (via drill 0.3)
  Top 0.254: v212.26,78.33 237.35,78.33 238.5,80.35 JP1.23
  Bottom 0.254: ENC4.B' 171.54,15.7 172.9,17.05 177.66,17.05 178.29,16.41 184.96,16.41 188.45,19.91 208.93,19.91 210.04,21.18 210.04,77.85 210.52,78.33 v212.26,78.33
  Bottom 0.406: R16.2 234.93,80.35 JP1.23
GPIO12  (via drill 0.3)
  Top 0.254: JP1.32 241.91,90.59 240.84,91.66 v220.84,91.66
  Bottom 0.254: ENC5.A' 223.27,115.36 222.43,114.52 222.43,108.49 223.06,107.86 223.06,104.05 220.84,101.5 v220.84,91.66
  Bottom 0.406: JP1.32 246.76,90.51 R17.2
GPIO13  (via drill 0.3)
  Top 0.254: v221.79,93.25 221.99,93.05 JP1.33
  Bottom 0.254: ENC5.B' 228.98,115.36 223.69,109.12 223.69,103.41 221.79,101.19 v221.79,93.25
  Bottom 0.406: JP1.33 234.92,93.05 R18.2
GPIO14
  Bottom 0.254: R63.1 C18.1 244.92,50.66 245.28,51.02 245.28,60.03
  Bottom 0.406: JP1.8 245.28,60.03 246.73,60.03 R19.2
GPIO15
  Top 0.254: JP2.5 245.81,56.85 244.33,58.33 244.33,61.3 243.06,62.57 JP1.10
  Bottom 0.254: IC2.20 279.85,75.51 280.53,74.83 280.53,58.64 278.94,57.05 270.45,57.05 JP2.5
  Bottom 0.406: R20.2 JP1.10
GPIO16  (via drill 0.3)
  Top 0.254: v212.9,93.41 213.06,93.73 213.53,94.2 240.53,94.2 JP1.36
  Bottom 0.254: ENC4.B 188.57,16.53 190.36,18.64 209.57,18.64 211.06,20.26 211.06,34.07 212.9,35.78 v212.9,93.41
  Bottom 0.406: R21.2 241.91,95.62 JP1.36
GPIO17  (via drill 0.2, 0.3)
  Top 0.254: JP1.11 239.46,65.11 240.84,63.72 244.97,63.72 245.28,63.41 v261.16,63.41 | v266.6,26.68 ENC1.A
  Bottom 0.254: v261.16,63.41 261.16,45.62 266.56,40.23 266.56,30.7 266.58,26.68 v266.6,26.68
  Bottom 0.305: R22.2
  Bottom 0.406: R22.2 JP1.11
GPIO18  (via drill 0.2, 0.3)
  Top 0.254: ENC1.B v267.52,24.09 | v262.11,64.04 245.72,64.04 244.65,65.11 JP1.12
  Bottom 0.254: v267.52,24.09 267.51,32.61 267.44,40.3 262.11,45.94 v262.11,64.04
  Bottom 0.406: R23.2 JP1.12
GPIO19  (via drill 0.3)
  Top 0.254: v216.39,24.35 217.34,25.3 217.34,31.66 v216.39,32.61 | v213.53,95.16 213.97,95.59 JP1.35
  Bottom 0.254: ENC4.A 189.22,10.51 190.36,11.65 190.36,16.41 191.79,18 209.72,18 v216.39,24.35 | v216.39,32.61 213.53,35.47 v213.53,95.16
  Bottom 0.406: JP1.35 R24.2
GPIO20
  Top 0.254: ENC2.B 78.07,15.75 80.44,18.12 119.21,18.12 121.51,15.82 126.92,15.82 129.06,17.96 175.89,17.96 178.36,15.49 184.88,15.49 188.68,19.28 209.17,19.28 210.61,20.72 210.61,96.44 210.91,96.74 240.84,96.74 241.91,97.82 JP1.38
  Bottom 0.406: R25.2 241.91,98.05 JP1.38
GPIO21  (via drill 0.3)
  Top 0.254: v218.46,102.3 219.25,102.46 240.12,102.46 JP1.40
  Bottom 0.254: ENC3.A 167.02,10.54 173.85,4.03 199.09,4.03 200.2,5.14 218.46,23.56 v218.46,102.3
  Bottom 0.406: R26.2 241.91,100.75 JP1.40
GPIO22  (via drill 0.3)
  Top 0.254: v64.54,4.08 v205.23,4.08 | v209.36,8.85 219.29,23.82 219.29,34.47 215.76,38.01 215.8,69.76 216.23,70.19 JP1.15
  Bottom 0.254: ENC2.E 63.57,15.71 61.8,17.23 59.74,17.27 59.02,16.4 59.02,9.29 v64.54,4.08 | v205.23,4.08 v209.36,8.85
  Bottom 0.305: R27.2
  Bottom 0.406: R27.2 JP1.15
GPIO23  (via drill 0.3)
  Top 0.254: v212.26,71.34 240.76,71.34 JP1.16
  Bottom 0.254: ENC4.E 185.01,15.51 188.61,19.27 209.25,19.27 210.55,20.7 210.68,69.75 v212.26,71.34
  Bottom 0.406: JP1.16 246.6,70.19 R28.2
GPIO24  (via drill 0.3)
  Top 0.254: JP1.18 241.68,72.73 240.52,73.88 v229.73,73.88
  Bottom 0.254: ENC5.E 229.14,101.14 230.61,99.92 230.61,96.86 230.5,96.75 230.36,74.52 v229.73,73.88
  Bottom 0.406: JP1.18 246.87,72.73 R29.2
GPIO25  (via drill 0.3)
  Top 0.254: JP1.22 241.91,78.2 240.84,79.28 240.84,81.19 240.52,81.5 237.98,81.5 236.71,82.77 v229.09,82.77
  Bottom 0.254: v229.09,82.77 229.09,98.29 ENC5.B
  Bottom 0.305: R30.2 246.71,77.81
  Bottom 0.406: 246.71,77.81 JP1.22
GPIO26
  Top 0.254: ENC2.A 76.9,10.57 75.66,11.81 75.66,17.12 77.2,18.66 119.54,18.66 121.71,16.5 126.75,16.5 128.81,18.56 176.19,18.56 178.43,16.33 184.88,16.33 185.03,16.48 185.08,16.48 188.46,19.86 208.79,19.86 210.06,21.12 210.06,98.01 211.97,99.92 233.54,99.92 235.33,98.13 JP1.37
  Bottom 0.406: JP1.37 234.92,98.13 R31.2
GPIO27  (via drill 0.3)
  Top 0.254: v221.11,67.65 JP1.13
  Bottom 0.254: ENC3.E 116.81,17.05 114.61,17.05 113.64,16.57 113.64,8.95 119.08,4.19 170.99,4.19 173.05,2.13 199.88,2.13 220.68,23.4 220.68,67.22 v221.11,67.65
  Bottom 0.305: R32.2 234.93,67.65
  Bottom 0.406: 234.93,67.65 JP1.13
N$1
  Bottom 1.422: X1.1 F1.1A
N$2
  Bottom 0.61: C2.1 20.3,58.77 20.5,58.96 | C1.1 17.76,58.77 17.95,58.96
  Bottom 1.016: 13.51,58.96 17.95,58.96 20.5,58.96 22.4,58.96 22.4,58.61 C3.1
  Bottom 1.422: F1.2A L1.P$1 13.51,64.03 13.51,58.96 13.07,58.52 D1.C
N$3
  Bottom 0.61: 13.95,72.39 13.95,71.86 14.78,71.03 17.95,71.03 | 17.95,71.03 20.5,71.03 20.5,69.52 R1.2 | C4.1 17.76,70.83 17.95,71.03 | 47K.2 17.76,71.22 17.95,71.03
  Bottom 1.422: Q1.2 13.95,72.39 L1.P$2
N$4
  Bottom 0.61: 17.32,75.47 15.93,76.86 Q2.3 11.63,78.62 10.97,79.28 10.97,79.61 Q1.1 | 17.32,75.47 20.14,75.47 C5.1 | 47K.1 17.76,75.03 17.32,75.47
N$5
  Bottom 0.61: C6.1 15.22,95.59 15.41,95.79 15.61,95.98 C8.1 | R3.2 18.15,95.59 17.95,95.79 | C9.1 18.79,95.98 18.59,95.79 | C10.1 21.96,95.98 21.77,95.79
  Bottom 1.016: 36.37,93.25 36.37,91.17 IC1.1
  Bottom 1.422: Q1.3 4.46,88.93 C14.+ 9.5,96.01 L2.P$1 11.41,97.89 13.51,95.79 15.41,95.79 17.95,95.79 18.59,95.79 21.77,95.79 33.83,95.79 36.37,93.25
N$6  (via drill 0.3)
  Top 0.254: S1.4 S1.3 20.99,97.72 21.06,97.66 16.01,97.66 15.49,97.14 15.49,78.08 v22.4,71.17
  Bottom 0.61: R1.1 21.97,67.42 22.4,67.85 22.4,71.12 v22.4,71.17 22.4,72.3 | 22.4,72.3 23.18,72.3 D2.1 | 22.4,72.3 21.32,72.3 C5.2
N$7
  Bottom 0.61: Q2.1 C7.1 16.68,83.88 | 16.68,83.88 18.11,83.88 56K.2 | C6.2 15.22,90.27 16.68,88.81 16.68,83.88
N$8
  Bottom 0.61: R3.1 18.15,86.31 56K.1 19.43,86.06 19.86,85.63 19.86,79.28 23.04,76.11 23.04,74.75 D2.2
N$9
  Bottom 0.61: 5.14,104.51 C11.1 C12.1
  Bottom 0.813: 5.14,104.51 6.67,104.51 6.84,104.68
  Bottom 1.422: L2.P$2 6.84,102.45 6.84,104.68 6.84,105.63 | 6.84,105.63 6.84,116.43 8.86,119.99 X2.4 | X2.1 10.89,105.63 6.84,105.63
N$10
  Bottom 1.016: IC1.2 39,89.35
  Bottom 1.422: 39,89.35 40.18,88.17 40.18,80.55 38.06,78.01 D3.C 34.69,63.08 L3.1
N$11
  Bottom 0.61: IC1.4 37.32,85.95 37.64,85.63 37.64,81.82 32.56,76.74 32.56,74.83 | C13.2 32.32,69.12 32.56,69.12 32.56,71.03 | 32.56,74.83 32.56,71.03 | R6.2 32.37,74.64 32.56,74.83 | R5.1 32.37,71.22 32.56,71.03
N$12
  Bottom 0.254: IC2.18 273.59,72.97 270.69,70.07 270.69,69.75 | 270.69,69.75 270.69,67.53 | 270.69,67.53 270.69,66.58 R49.1 | C17.1 270.49,67.73 270.69,67.53 | C16.2 270.56,69.88 270.69,69.75
N$13
  Bottom 0.254: R59.1 R55.2 287.05,112.45 T1.1
N$14
  Bottom 0.61: R50.1 20.77,116.02 LED1.A
N$15
  Bottom 0.254: R60.1 R56.2 269.88,112.45 T2.1
N$16
  Bottom 0.254: R51.2 241.22,117.26 LED2.A
N$17
  Bottom 0.254: LED3.A 259.24,114.53 257.35,116.43 256.18,116.43 R52.2
N$18
  Bottom 0.254: R53.2 275.18,116.94 LED4.A
N$19
  Bottom 0.254: R54.2 292.37,116.94 LED5.A
N$20
  Bottom 0.254: R61.1 R57.2 252.1,111.77 T3.1
N$21
  Bottom 0.254: R62.1 R58.2 238.3,112.94 238.62,112.61 T4.1
N$22
  Bottom 0.254: T1.3 292.75,110.25 292.75,113.5 R54.1
N$23
  Bottom 0.254: JP5.2 267.62,119.49 268.78,118.33 285.61,118.33 R59.2
N$24
  Bottom 0.254: R60.2 267.19,116.74 264.97,118.97 264.97,120.32 JP5.3
N$25
  Bottom 0.254: JP5.4 262.55,119.08 261.8,118.33 252.59,118.33 251.95,117.7 R61.2
N$26
  Bottom 0.254: JP5.5 238.5,120.43 236.71,118.65 R62.2
N$27
  Bottom 0.254: T2.3 275.25,110.25 275.5,110.5 275.5,113.6 R53.1
N$28
  Bottom 0.254: T3.3 257.45,110.2 257.5,110.25 257.5,113.49 R52.1
N$29
  Bottom 0.254: T4.3 241.75,110.25 241.75,114.01 R51.1
N$30
  Top 0.406: TR2.6 64.35,37 JP8.1
N$31
  Top 0.406: TR2.4 54.19,37 JP8.2
N$32
  Bottom 0.254: R64.1 R63.2
N$33
  Bottom 0.254: JP6.1 R64.2
N$34
  Top 0.406: R83.E 69.54,69.14 R75.1
N$35
  Top 0.406: C23.+ 62.27,58.65 R83.A R83.S
N$37  (via drill 0.8 pad 1.93)
  other vias: 80.82,117.38
N$38  (via drill 0.8 pad 1.93)
  other vias: 80.82,114.84
N$39  (via drill 0.8 pad 1.93)
  other vias: 80.82,112.3
N$40  (via drill 0.8 pad 1.93)
  other vias: 80.82,109.76
N$41  (via drill 0.8 pad 1.93)
  other vias: 80.82,107.22
N$42  (via drill 0.8 pad 1.93)
  other vias: 80.82,104.68
N$43  (via drill 0.8 pad 1.93)
  other vias: 80.82,102.14
N$44  (via drill 0.8 pad 1.93)
  other vias: 80.82,99.6
N$45  (via drill 0.8 pad 1.93)
  other vias: 80.82,97.06
N$46  (via drill 0.8 pad 1.93)
  other vias: 80.82,94.52
N$47  (via drill 0.8 pad 1.93)
  other vias: 80.82,91.98
N$48  (via drill 0.8 pad 1.93)
  other vias: 80.82,89.44
N$49  (via drill 0.8 pad 1.93)
  other vias: 80.82,86.9
N$50  (via drill 0.8 pad 1.93)
  other vias: 80.82,84.36
N$51  (via drill 0.8 pad 1.93)
  other vias: 80.82,81.82
N$52  (via drill 0.8 pad 1.93)
  other vias: 80.82,79.28
N$53  (via drill 0.8 pad 1.93)
  other vias: 80.82,76.74
N$54  (via drill 0.8 pad 1.93)
  other vias: 80.82,74.2
N$55  (via drill 0.8 pad 1.93)
  other vias: 80.82,71.66
N$56  (via drill 0.8 pad 1.93)
  other vias: 80.82,69.12
N$57  (via drill 0.8 pad 1.93)
  other vias: 80.82,66.58
N$58  (via drill 0.8 pad 1.93)
  other vias: 80.82,64.04
N$59  (via drill 0.8 pad 1.93)
  other vias: 80.82,61.5
N$60  (via drill 0.8 pad 1.93)
  other vias: 80.82,58.96
N$61  (via drill 0.8 pad 1.93)
  other vias: 80.82,56.42
N$62  (via drill 0.8 pad 1.93)
  other vias: 80.82,53.88
N$63  (via drill 0.8 pad 1.93)
  other vias: 80.82,51.34
N$64  (via drill 0.8 pad 1.93)
  other vias: 80.82,48.8
N$65  (via drill 0.8 pad 1.93)
  other vias: 80.82,46.26
N$66  (via drill 0.8 pad 1.93)
  other vias: 80.82,43.72
N$67  (via drill 0.8 pad 1.93)
  other vias: 80.82,41.18
N$68  (via drill 0.8 pad 1.93)
  other vias: 80.82,38.64
N$69  (via drill 0.8 pad 1.93)
  other vias: 80.82,36.1
N$70  (via drill 0.8 pad 1.93)
  other vias: 80.82,33.56
N$71  (via drill 0.8 pad 1.93)
  other vias: 80.82,31.02
N$72  (via drill 0.8 pad 1.93)
  other vias: 80.82,28.48
N$77  (via drill 0.8 pad 1.93)
  other vias: 78.28,114.84
N$78  (via drill 0.8 pad 1.93)
  other vias: 78.28,112.3
N$79  (via drill 0.8 pad 1.93)
  other vias: 78.28,109.76
N$80  (via drill 0.8 pad 1.93)
  other vias: 78.28,107.22
N$81  (via drill 0.8 pad 1.93)
  other vias: 78.28,104.68
N$82  (via drill 0.8 pad 1.93)
  other vias: 78.28,102.14
N$83  (via drill 0.8 pad 1.93)
  other vias: 78.28,99.6
N$84  (via drill 0.8 pad 1.93)
  other vias: 78.28,97.06
N$85  (via drill 0.8 pad 1.93)
  other vias: 78.28,94.52
N$86  (via drill 0.8 pad 1.93)
  other vias: 78.28,91.98
N$87  (via drill 0.8 pad 1.93)
  other vias: 78.28,89.44
N$88  (via drill 0.8 pad 1.93)
  other vias: 78.28,86.9
N$89  (via drill 0.8 pad 1.93)
  other vias: 78.28,84.36
N$90  (via drill 0.8 pad 1.93)
  other vias: 78.28,81.82
N$91  (via drill 0.8 pad 1.93)
  other vias: 78.28,79.28
N$92  (via drill 0.8 pad 1.93)
  other vias: 78.28,76.74
N$93  (via drill 0.8 pad 1.93)
  other vias: 78.28,74.2
N$94  (via drill 0.8 pad 1.93)
  other vias: 78.28,71.66
N$95  (via drill 0.8 pad 1.93)
  other vias: 78.28,69.12
N$96
  Top 0.406: R70.2 Q9.3 62.48,86.19 63.67,85 63.67,79.92 63.04,79.28 62.41,79.28 Q11.B
N$97  (via drill 0.2)
  Top 0.406: Q11.E 62.37,82.42 v62.41,82.45 | v54.78,82.45 53.52,82.45 | 53.52,82.45 53.52,85.63 | 53.52,85.63 52.78,85.63 R69.2 | R70.1 54.08,86.19 53.52,85.63 | 53.52,82.45 52.22,81.16 R76.2 53.34,78.19 54.78,76.74 54.78,74.55 IC6.3
  Bottom 0.406: v62.41,82.45 v54.78,82.45
N$98
  Top 0.406: C22.- 67.27,103.19 66.22,102.14 66.22,99.3 C20.2 | C24.1 C20.2 | C20.2 R66.2 R68.2
N$99  (via drill 0.2)
  Top 0.406: Q9.2 Q11.C 60.17,78.34 v60.5,78.01 | R75.2 67.95,72.41 R73.1 67.84,72.3 v66.22,72.3
  Bottom 0.406: v60.5,78.01 v66.22,72.3
N$100
  Top 0.406: R67.1 60.22,87.19 Q9.1
N$101
  Top 0.406: C21.- 58.27,99.24 C19.1 | C19.1 C24.2 | C19.1 R65.2 58.22,93.29 R67.2
N$102
  Top 0.406: R68.1 68.22,87.19 Q10.1
N$103  (via drill 0.2)
  Top 0.406: Q12.E 70.37,82.11 v70.03,82.45 | v53.52,87.53 53.52,88.81 | 53.52,88.81 52.59,88.81 R71.2 | R72.1 53.9,89.19 53.52,88.81 | IC6.2 56.17,76.22 56.69,76.74 60.5,76.74 61.14,76.11 | 61.14,76.11 61.14,72.72 R77.2 | 61.14,76.11 61.77,76.11 64.94,79.28 v64.94,85.63
  Bottom 0.406: v70.03,82.45 68.12,82.45 v64.94,85.63 63.04,87.53 v53.52,87.53
N$104  (via drill 0.2)
  Top 0.406: v64.31,88.81 66.92,86.19 Q10.3 70.73,86.19 71.93,85 71.93,79.92 71.3,79.28 70.41,79.28 Q12.B | v58.59,88.81 57.6,88.81 R72.2
  Bottom 0.406: v64.31,88.81 v58.59,88.81
N$105
  Top 0.406: Q10.2 Q12.C 68.17,75.42 R74.1 63.39,75.19 63.04,74.83 63.04,66.5 C23.-
N$106  (via drill 0.8 pad 1.93)
  other vias: 78.28,66.58
N$107
  Top 0.406: IC6.6 54.91,67.22 | 54.91,67.22 54.91,65.09 C25.+ | R77.1 61.17,67.89 60.5,67.22 54.91,67.22
N$108  (via drill 0.8 pad 1.93)
  other vias: 78.28,64.04
N$109  (via drill 0.8 pad 1.93)
  other vias: 78.28,61.5
N$110
  Top 0.406: JP15.3 61.14,113.19 61.14,109.76 C21.+
N$111
  Top 0.406: JP15.1 66.08,108.65 C22.+
N$112
  Top 0.406: R78.2 49,60.83 C25.- 54.7,60.83 TR2.1
N$113  (via drill 0.8 pad 1.93)
  other vias: 78.28,58.96
N$114  (via drill 0.8 pad 1.93)
  other vias: 78.28,56.42
N$115  (via drill 0.8 pad 1.93)
  other vias: 78.28,53.88
N$116  (via drill 0.8 pad 1.93)
  other vias: 78.28,51.34
N$117  (via drill 0.8 pad 1.93)
  other vias: 78.28,48.8
N$118  (via drill 0.8 pad 1.93)
  other vias: 78.28,46.26
N$119  (via drill 0.8 pad 1.93)
  other vias: 78.28,43.72
N$120  (via drill 0.8 pad 1.93)
  other vias: 78.28,41.18
N$121  (via drill 0.8 pad 1.93)
  other vias: 78.28,38.64
N$122  (via drill 0.8 pad 1.93)
  other vias: 78.28,36.1
N$123  (via drill 0.8 pad 1.93)
  other vias: 78.28,33.56
N$124  (via drill 0.8 pad 1.93)
  other vias: 78.28,31.02
N$128  (via drill 0.8 pad 1.93)
  other vias: 83.36,119.92
N$129  (via drill 0.8 pad 1.93)
  other vias: 83.36,117.38
N$130  (via drill 0.8 pad 1.93)
  other vias: 83.36,114.84
N$131  (via drill 0.8 pad 1.93)
  other vias: 83.36,112.3
N$132  (via drill 0.8 pad 1.93)
  other vias: 83.36,109.76
N$133  (via drill 0.8 pad 1.93)
  other vias: 83.36,107.22
N$134  (via drill 0.8 pad 1.93)
  other vias: 83.36,104.68
N$135  (via drill 0.8 pad 1.93)
  other vias: 83.36,102.14
N$136  (via drill 0.8 pad 1.93)
  other vias: 83.36,99.6
N$137  (via drill 0.8 pad 1.93)
  other vias: 83.36,97.06
N$138  (via drill 0.8 pad 1.93)
  other vias: 83.36,94.52
N$139  (via drill 0.8 pad 1.93)
  other vias: 83.36,91.98
N$140  (via drill 0.8 pad 1.93)
  other vias: 83.36,89.44
N$141  (via drill 0.8 pad 1.93)
  other vias: 83.36,86.9
N$142  (via drill 0.8 pad 1.93)
  other vias: 83.36,84.36
N$143  (via drill 0.8 pad 1.93)
  other vias: 83.36,81.82
N$144  (via drill 0.8 pad 1.93)
  other vias: 83.36,79.28
N$145  (via drill 0.8 pad 1.93)
  other vias: 83.36,76.74
N$146  (via drill 0.8 pad 1.93)
  other vias: 83.36,74.2
N$147  (via drill 0.8 pad 1.93)
  other vias: 83.36,71.66
N$148  (via drill 0.8 pad 1.93)
  other vias: 83.36,69.12
N$149
  Top 0.406: R80.1 R79.2
N$150
  Top 0.406: JP15.4 51.32,113.19 R80.2
N$151  (via drill 0.8 pad 1.93)
  other vias: 83.36,66.58
N$152  (via drill 0.8 pad 1.93)
  other vias: 83.36,64.04
N$153  (via drill 0.8 pad 1.93)
  other vias: 83.36,61.5
N$154  (via drill 0.8 pad 1.93)
  other vias: 83.36,58.96
N$155  (via drill 0.8 pad 1.93)
  other vias: 83.36,56.42
N$156  (via drill 0.8 pad 1.93)
  other vias: 83.36,53.88
N$157  (via drill 0.8 pad 1.93)
  other vias: 83.36,51.34
N$158  (via drill 0.8 pad 1.93)
  other vias: 83.36,48.8
N$159  (via drill 0.8 pad 1.93)
  other vias: 83.36,46.26
N$160  (via drill 0.8 pad 1.93)
  other vias: 83.36,43.72
N$161  (via drill 0.8 pad 1.93)
  other vias: 83.36,41.18
N$162  (via drill 0.8 pad 1.93)
  other vias: 83.36,38.64
N$163  (via drill 0.8 pad 1.93)
  other vias: 83.36,36.1
N$164  (via drill 0.8 pad 1.93)
  other vias: 83.36,33.56
N$165  (via drill 0.8 pad 1.93)
  other vias: 83.36,31.02
N$166  (via drill 0.8 pad 1.93)
  other vias: 83.36,28.48
N$167  (via drill 0.8 pad 1.93)
  other vias: 83.36,25.94
N$169  (via drill 0.8 pad 1.93)
  other vias: 85.9,119.92
N$170  (via drill 0.8 pad 1.93)
  other vias: 85.9,117.38
N$171  (via drill 0.8 pad 1.93)
  other vias: 85.9,114.84
N$172  (via drill 0.8 pad 1.93)
  other vias: 85.9,112.3
N$173  (via drill 0.8 pad 1.93)
  other vias: 85.9,109.76
N$174  (via drill 0.8 pad 1.93)
  other vias: 85.9,107.22
N$175  (via drill 0.8 pad 1.93)
  other vias: 85.9,104.68
N$176  (via drill 0.8 pad 1.93)
  other vias: 85.9,102.14
N$177  (via drill 0.8 pad 1.93)
  other vias: 85.9,99.6
N$178  (via drill 0.8 pad 1.93)
  other vias: 85.9,97.06
N$179  (via drill 0.8 pad 1.93)
  other vias: 85.9,94.52
N$180  (via drill 0.8 pad 1.93)
  other vias: 85.9,91.98
N$181  (via drill 0.8 pad 1.93)
  other vias: 85.9,89.44
N$182  (via drill 0.8 pad 1.93)
  other vias: 85.9,86.9
N$183  (via drill 0.8 pad 1.93)
  other vias: 85.9,84.36
N$184  (via drill 0.8 pad 1.93)
  other vias: 85.9,81.82
N$185  (via drill 0.8 pad 1.93)
  other vias: 85.9,79.28
N$186  (via drill 0.8 pad 1.93)
  other vias: 85.9,76.74
N$187  (via drill 0.8 pad 1.93)
  other vias: 85.9,74.2
N$188  (via drill 0.8 pad 1.93)
  other vias: 85.9,71.66
N$189  (via drill 0.8 pad 1.93)
  other vias: 85.9,69.12
N$190  (via drill 0.8 pad 1.93)
  other vias: 85.9,66.58
N$191  (via drill 0.8 pad 1.93)
  other vias: 85.9,64.04
N$192  (via drill 0.8 pad 1.93)
  other vias: 85.9,61.5
N$193  (via drill 0.8 pad 1.93)
  other vias: 85.9,58.96
N$194  (via drill 0.8 pad 1.93)
  other vias: 85.9,56.42
N$195  (via drill 0.8 pad 1.93)
  other vias: 85.9,53.88
N$196  (via drill 0.8 pad 1.93)
  other vias: 85.9,51.34
N$197  (via drill 0.8 pad 1.93)
  other vias: 85.9,48.8
N$198  (via drill 0.8 pad 1.93)
  other vias: 85.9,46.26
N$199  (via drill 0.8 pad 1.93)
  other vias: 85.9,43.72
N$200  (via drill 0.8 pad 1.93)
  other vias: 85.9,41.18
N$201  (via drill 0.8 pad 1.93)
  other vias: 85.9,38.64
N$202  (via drill 0.8 pad 1.93)
  other vias: 85.9,36.1
N$203  (via drill 0.8 pad 1.93)
  other vias: 85.9,33.56
N$204  (via drill 0.8 pad 1.93)
  other vias: 85.9,31.02
N$205  (via drill 0.8 pad 1.93)
  other vias: 85.9,28.48
N$206  (via drill 0.8 pad 1.93)
  other vias: 85.9,25.94
N$208  (via drill 0.8 pad 1.93)
  other vias: 88.44,119.92
N$209  (via drill 0.8 pad 1.93)
  other vias: 88.44,117.38
N$210  (via drill 0.8 pad 1.93)
  other vias: 88.44,114.84
N$211  (via drill 0.8 pad 1.93)
  other vias: 88.44,112.3
N$212  (via drill 0.8 pad 1.93)
  other vias: 88.44,109.76
N$213  (via drill 0.8 pad 1.93)
  other vias: 88.44,107.22
N$214  (via drill 0.8 pad 1.93)
  other vias: 88.44,104.68
N$215  (via drill 0.8 pad 1.93)
  other vias: 88.44,102.14
N$216  (via drill 0.8 pad 1.93)
  other vias: 88.44,99.6
N$217  (via drill 0.8 pad 1.93)
  other vias: 88.44,97.06
N$218  (via drill 0.8 pad 1.93)
  other vias: 88.44,94.52
N$219  (via drill 0.8 pad 1.93)
  other vias: 88.44,91.98
N$220  (via drill 0.8 pad 1.93)
  other vias: 88.44,89.44
N$221  (via drill 0.8 pad 1.93)
  other vias: 88.44,86.9
N$222  (via drill 0.8 pad 1.93)
  other vias: 88.44,84.36
N$223  (via drill 0.8 pad 1.93)
  other vias: 88.44,81.82
N$224  (via drill 0.8 pad 1.93)
  other vias: 88.44,79.28
N$225  (via drill 0.8 pad 1.93)
  other vias: 88.44,76.74
N$226  (via drill 0.8 pad 1.93)
  other vias: 88.44,74.2
N$227  (via drill 0.8 pad 1.93)
  other vias: 88.44,71.66
N$228  (via drill 0.8 pad 1.93)
  other vias: 88.44,69.12
N$229  (via drill 0.8 pad 1.93)
  other vias: 88.44,66.58
N$230  (via drill 0.8 pad 1.93)
  other vias: 88.44,64.04
N$231  (via drill 0.8 pad 1.93)
  other vias: 88.44,61.5
N$232  (via drill 0.8 pad 1.93)
  other vias: 88.44,58.96
N$233  (via drill 0.8 pad 1.93)
  other vias: 88.44,56.42
N$234  (via drill 0.8 pad 1.93)
  other vias: 88.44,53.88
N$235  (via drill 0.8 pad 1.93)
  other vias: 88.44,51.34
N$236  (via drill 0.8 pad 1.93)
  other vias: 88.44,48.8
N$237  (via drill 0.8 pad 1.93)
  other vias: 88.44,46.26
N$238  (via drill 0.8 pad 1.93)
  other vias: 88.44,43.72
N$239  (via drill 0.8 pad 1.93)
  other vias: 88.44,41.18
N$240  (via drill 0.8 pad 1.93)
  other vias: 88.44,38.64
N$241  (via drill 0.8 pad 1.93)
  other vias: 88.44,36.1
N$242  (via drill 0.8 pad 1.93)
  other vias: 88.44,33.56
N$243  (via drill 0.8 pad 1.93)
  other vias: 88.44,31.02
N$244  (via drill 0.8 pad 1.93)
  other vias: 88.44,28.48
N$245  (via drill 0.8 pad 1.93)
  other vias: 88.44,25.94
N$247  (via drill 0.8 pad 1.93)
  other vias: 90.98,119.92
N$248  (via drill 0.8 pad 1.93)
  other vias: 90.98,117.38
N$249  (via drill 0.8 pad 1.93)
  other vias: 90.98,114.84
N$250  (via drill 0.8 pad 1.93)
  other vias: 90.98,112.3
N$251  (via drill 0.8 pad 1.93)
  other vias: 90.98,109.76
N$252  (via drill 0.8 pad 1.93)
  other vias: 90.98,107.22
N$253  (via drill 0.8 pad 1.93)
  other vias: 90.98,104.68
N$254  (via drill 0.8 pad 1.93)
  other vias: 90.98,102.14
N$255  (via drill 0.8 pad 1.93)
  other vias: 90.98,99.6
N$256  (via drill 0.8 pad 1.93)
  other vias: 90.98,97.06
N$257  (via drill 0.8 pad 1.93)
  other vias: 90.98,94.52
N$258  (via drill 0.8 pad 1.93)
  other vias: 90.98,91.98
N$259  (via drill 0.8 pad 1.93)
  other vias: 90.98,89.44
N$260  (via drill 0.8 pad 1.93)
  other vias: 90.98,86.9
N$261  (via drill 0.8 pad 1.93)
  other vias: 90.98,84.36
N$262  (via drill 0.8 pad 1.93)
  other vias: 90.98,81.82
N$263  (via drill 0.8 pad 1.93)
  other vias: 90.98,79.28
N$264  (via drill 0.8 pad 1.93)
  other vias: 90.98,76.74
N$265  (via drill 0.8 pad 1.93)
  other vias: 90.98,74.2
N$266  (via drill 0.8 pad 1.93)
  other vias: 90.98,71.66
N$267  (via drill 0.8 pad 1.93)
  other vias: 90.98,69.12
N$268  (via drill 0.8 pad 1.93)
  other vias: 90.98,66.58
N$269  (via drill 0.8 pad 1.93)
  other vias: 90.98,64.04
N$270  (via drill 0.8 pad 1.93)
  other vias: 90.98,61.5
N$271  (via drill 0.8 pad 1.93)
  other vias: 90.98,58.96
N$272  (via drill 0.8 pad 1.93)
  other vias: 90.98,56.42
N$273  (via drill 0.8 pad 1.93)
  other vias: 90.98,53.88
N$274  (via drill 0.8 pad 1.93)
  other vias: 90.98,51.34
N$275  (via drill 0.8 pad 1.93)
  other vias: 90.98,48.8
N$276  (via drill 0.8 pad 1.93)
  other vias: 90.98,46.26
N$277  (via drill 0.8 pad 1.93)
  other vias: 90.98,43.72
N$278  (via drill 0.8 pad 1.93)
  other vias: 90.98,41.18
N$279  (via drill 0.8 pad 1.93)
  other vias: 90.98,38.64
N$280  (via drill 0.8 pad 1.93)
  other vias: 90.98,36.1
N$281  (via drill 0.8 pad 1.93)
  other vias: 90.98,33.56
N$282  (via drill 0.8 pad 1.93)
  other vias: 90.98,31.02
N$283  (via drill 0.8 pad 1.93)
  other vias: 90.98,28.48
N$284  (via drill 0.8 pad 1.93)
  other vias: 90.98,25.94
N$286  (via drill 0.8 pad 1.93)
  other vias: 93.52,119.92
N$287  (via drill 0.8 pad 1.93)
  other vias: 93.52,117.38
N$288  (via drill 0.8 pad 1.93)
  other vias: 93.52,114.84
N$289  (via drill 0.8 pad 1.93)
  other vias: 93.52,112.3
N$290  (via drill 0.8 pad 1.93)
  other vias: 93.52,109.76
N$291  (via drill 0.8 pad 1.93)
  other vias: 93.52,107.22
N$292  (via drill 0.8 pad 1.93)
  other vias: 93.52,104.68
N$293  (via drill 0.8 pad 1.93)
  other vias: 93.52,102.14
N$294  (via drill 0.8 pad 1.93)
  other vias: 93.52,99.6
N$295  (via drill 0.8 pad 1.93)
  other vias: 93.52,97.06
N$296  (via drill 0.8 pad 1.93)
  other vias: 93.52,94.52
N$297  (via drill 0.8 pad 1.93)
  other vias: 93.52,91.98
N$298  (via drill 0.8 pad 1.93)
  other vias: 93.52,89.44
N$299  (via drill 0.8 pad 1.93)
  other vias: 93.52,86.9
N$300  (via drill 0.8 pad 1.93)
  other vias: 93.52,84.36
N$301  (via drill 0.8 pad 1.93)
  other vias: 93.52,81.82
N$302  (via drill 0.8 pad 1.93)
  other vias: 93.52,79.28
N$303  (via drill 0.8 pad 1.93)
  other vias: 93.52,76.74
N$304  (via drill 0.8 pad 1.93)
  other vias: 93.52,74.2
N$305  (via drill 0.8 pad 1.93)
  other vias: 93.52,71.66
N$306  (via drill 0.8 pad 1.93)
  other vias: 93.52,69.12
N$307  (via drill 0.8 pad 1.93)
  other vias: 93.52,66.58
N$308  (via drill 0.8 pad 1.93)
  other vias: 93.52,64.04
N$309  (via drill 0.8 pad 1.93)
  other vias: 93.52,61.5
N$310  (via drill 0.8 pad 1.93)
  other vias: 93.52,58.96
N$311  (via drill 0.8 pad 1.93)
  other vias: 93.52,56.42
N$312  (via drill 0.8 pad 1.93)
  other vias: 93.52,53.88
N$313  (via drill 0.8 pad 1.93)
  other vias: 93.52,51.34
N$314  (via drill 0.8 pad 1.93)
  other vias: 93.52,48.8
N$315  (via drill 0.8 pad 1.93)
  other vias: 93.52,46.26
N$316  (via drill 0.8 pad 1.93)
  other vias: 93.52,43.72
N$317  (via drill 0.8 pad 1.93)
  other vias: 93.52,41.18
N$318  (via drill 0.8 pad 1.93)
  other vias: 93.52,38.64
N$319  (via drill 0.8 pad 1.93)
  other vias: 93.52,36.1
N$320  (via drill 0.8 pad 1.93)
  other vias: 93.52,33.56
